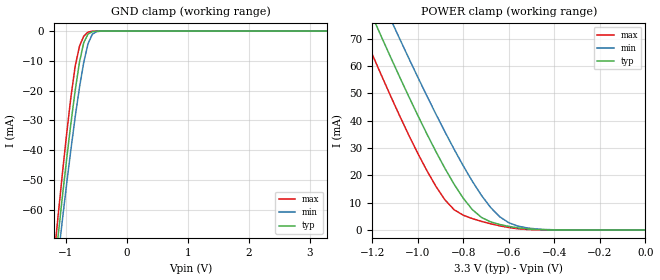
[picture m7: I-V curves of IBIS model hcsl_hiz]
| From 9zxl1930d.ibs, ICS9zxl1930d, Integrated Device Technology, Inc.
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|   Model hcsl_hiz
[Model]  hcsl_hiz
Model_type Input
Polarity   Non-Inverting
Vinl =   0.8000V
Vinh =   2.0000V
C_comp   2.8800pF   2.8800pF   2.8800pF
[Temperature Range]   25.0000   85.0000   -40.0000
[Voltage Range]   3.3000V   3.1350V   3.4650V
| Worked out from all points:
|   GND clamp passes 1 mA (typ) near -0.64 V on its own axis
|   POWER clamp passes 1 mA (typ) near -0.58 V on its own axis
[GND_clamp]
|Voltage   I(typ)   I(min)   I(max)
-3.3V     -538.1mA   -521.5mA   -558.6mA
-1.2V     -82.49mA   -88.9mA    -76.63mA
-1.13V    -68.87mA   -76.02mA   -62.04mA
-1.06V    -55.67mA   -63.48mA   -47.95mA
-920mV    -30.99mA   -39.77mA   -22.19mA
-850mV    -19.96mA   -28.87mA   -11.8mA
-780mV    -10.51mA   -18.98mA   -5.147mA
-710mV    -3.897mA   -10.54mA   -1.703mA
-640mV    -1.025mA   -4.296mA   -353.9uA
-570mV    -215.5uA   -1.07mA    -49.96uA
-430mV    -5.64uA    -33.89uA   -409.2nA
3.28V     309.8pA    62.52nA    311pA
[POWER_clamp]
|Voltage   I(typ)   I(min)   I(max)
-3.28V    519.3mA    524.5mA    517.5mA
-1.28V    93.7mA     107.1mA    80.13mA
-1.24V    86.01mA    99.59mA    72.23mA
-1.16V    70.88mA    84.72mA    56.77mA
-1.12V    63.47mA    77.4mA     49.26mA
-1.08V    56.18mA    70.18mA    41.94mA
-960mV    35.23mA    49.16mA    21.78mA
-880mV    22.49mA    35.88mA    10.99mA
-760mV    7.449mA    17.82mA    4.155mA
-640mV    2.007mA    4.846mA    1.512mA
-480mV    168.9uA    373.5uA    48.5uA
0V        320pA      624.8pA    341.5pA
